| TEXAS INSTRUMENTS INCORPORATED
| Standard Linear and Logic Group
| IBIS Model of SN74LVC14A
| HEX SCHMITT-TRIGGER INVERTERS
| This file contains package information for the following:
|  SOIC 14-pin (D) package as [Component] LVC14A_D
|  SSOP 14-pin (DB) package as [Component] LVC14A_DB
|  TVSOP 14-pin (DGV) package as [Component] LVC14A_DGV
|  SOP 14-pin (NS) package as [Component] LVC14A_NS
|  TSSOP 14-pin (PW) package as [Component] LVC14A_PW
|  QFN 14-pin (RGY) package as [Component] LVC14A_RGY
| This device can be powered at the following Vccs:
|  1.8 volt Vcc
|  2.5 volt Vcc
|  3.3 volt Vcc
|  2.7 volt Vcc
| This file provides unique models under the [Model Selector] for each Vcc.
| For operation at a specific Vcc, select the appropriate model after each
| [Model Selector] keyword.
[IBIS Ver]   3.2
[Comment char]  |_char
[File Name]   sn74lvc14a.ibs
[File Rev]   1.1 | k_die
[Date]   March 31, 2004
[Source]   Data created from TI-SPICE simulations at TI-SLL.
[Notes]   The following is an IBIS list for the LVC14A.
   Please contact sllibis@ti.com with questions and
   comments concerning SLL IBIS models.
   - FILE REV HISTORY
   - 1.1 Release IBIS file on 04/01/04
   - Power clamp data deleted as there is no power-clamp diode.
[Disclaimer] Property of Texas Instruments Incorporated.  Unauthorized
   reproduction and/or distribution is strictly prohibited.
   This product is protected under copyright law.
   Created  2004, (C) Copyright  2004, Texas Instruments
   Incorporated, All Rights Reserved
   UNLESS THERE IS A SIGNED, WRITTEN AGREEMENT TO THE
   CONTRARY, TEXAS INSTRUMENTS (TI) IS PROVIDING THE IBIS
   MODELS  AND WITHOUT ANY WARRANTY, EXPRESSED OR
   IMPLIED.  TI assumes no liability for:
   1) the accuracy of the IBIS models provided to your
   company;
   2) the proper functioning of these IBIS Models in your
   design or for any resulting applications; or
   3) infringement of patents, copyrights or intellectual
   property rights resulting from your use of these IBIS
   models.
   TI provides IBIS Models as a service to our customers.
   You and your company shall not distribute, sell or give
   these models to anyone else without prior written
   permission from TI.
   TI reserves the right to make changes to our products or
   to discontinue any semiconductor product or service
   without notice, and advises our customers to obtain the
   latest version of relevant information to verify, before
   placing orders, that the information being relied on is
   current.
   Please be aware that your receipt and use of the IBIS
   information provided shall serve as acceptance of these
   terms and conditions.  If you do not accept these terms,
   you should return or destroy the IBIS models and any
   other accompanying information immediately.
| Component LVC14A_D 14-pin SOIC
[Component]   LVC14A_D
[Manufacturer]   Texas Instruments, Inc.
[Package]
|   typ   min   max
R_pkg   3.100e-02   2.800e-02   3.400e-02
L_pkg   3.109e-09   2.462e-09   3.889e-09
C_pkg   4.730e-13   3.630e-13   6.280e-13
[Pin]   signal_name   model_name   R_pin   L_pin   C_pin
1   1A   LVC14A_IN   3.300e-02   3.854e-09   6.220e-13
2   1Y   LVC14A_OUT   3.200e-02   3.188e-09   4.730e-13
3   2A   LVC14A_IN   2.800e-02   2.462e-09   3.770e-13
4   2Y   LVC14A_OUT   3.100e-02   2.596e-09   3.630e-13
5   3A   LVC14A_IN   2.800e-02   2.521e-09   3.720e-13
6   3Y   LVC14A_OUT   3.400e-02   3.250e-09   4.760e-13
7   GND   GND   3.400e-02   3.889e-09   6.280e-13
8   4Y   LVC14A_OUT   3.400e-02   3.889e-09   6.280e-13
9   4A   LVC14A_IN   3.400e-02   3.250e-09   4.760e-13
10   5Y   LVC14A_OUT   2.800e-02   2.521e-09   3.720e-13
11   5A   LVC14A_IN   3.100e-02   2.596e-09   3.640e-13
12   6Y   LVC14A_OUT   2.800e-02   2.462e-09   3.770e-13
13   6A   LVC14A_IN   3.200e-02   3.188e-09   4.730e-13
14   VCC   POWER   3.300e-02   3.854e-09   6.220e-13
| Component LVC14A_DB 14-pin SSOP
[Component]   LVC14A_DB
[Manufacturer]   Texas Instruments, Inc.
[Package]
|   typ   min   max
R_pkg   4.400e-02   4.100e-02   4.600e-02
L_pkg   3.551e-09   3.258e-09   3.927e-09
C_pkg   4.020e-13   3.600e-13   4.210e-13
[Pin]   signal_name   model_name   R_pin   L_pin   C_pin
1   1A   LVC14A_IN   4.600e-02   3.927e-09   4.080e-13
2   1Y   LVC14A_OUT   4.400e-02   3.587e-09   4.210e-13
3   2A   LVC14A_IN   4.100e-02   3.289e-09   3.980e-13
4   2Y   LVC14A_OUT   4.200e-02   3.258e-09   3.600e-13
5   3A   LVC14A_IN   4.100e-02   3.286e-09   4.030e-13
6   3Y   LVC14A_OUT   4.400e-02   3.586e-09   4.210e-13
7   GND   GND   4.600e-02   3.927e-09   4.080e-13
8   4Y   LVC14A_OUT   4.600e-02   3.927e-09   4.080e-13
9   4A   LVC14A_IN   4.400e-02   3.586e-09   4.210e-13
10   5Y   LVC14A_OUT   4.100e-02   3.286e-09   4.030e-13
11   5A   LVC14A_IN   4.300e-02   3.258e-09   3.600e-13
12   6Y   LVC14A_OUT   4.100e-02   3.289e-09   3.980e-13
13   6A   LVC14A_IN   4.400e-02   3.587e-09   4.210e-13
14   VCC   POWER   4.600e-02   3.927e-09   4.080e-13
| Component LVC14A_DGV 14-pin TVSOP
[Component]   LVC14A_DGV
[Manufacturer]   Texas Instruments, Inc.
[Package]
|   typ   min   max
R_pkg   3.500e-02   2.000e-02   4.500e-02
L_pkg   2.499e-09   2.077e-09   2.966e-09
C_pkg   3.610e-13   3.050e-13   4.160e-13
[Pin]   signal_name   model_name   R_pin   L_pin   C_pin
1   1A   LVC14A_IN   2.700e-02   2.717e-09   3.730e-13
2   1Y   LVC14A_OUT   3.700e-02   2.434e-09   3.980e-13
3   2A   LVC14A_IN   3.400e-02   2.200e-09   3.160e-13
4   2Y   LVC14A_OUT   2.000e-02   2.077e-09   3.090e-13
5   3A   LVC14A_IN   3.000e-02   2.147e-09   3.050e-13
6   3Y   LVC14A_OUT   4.200e-02   2.580e-09   4.080e-13
7   GND   GND   3.900e-02   2.921e-09   3.850e-13
8   4Y   LVC14A_OUT   3.300e-02   2.841e-09   3.800e-13
9   4A   LVC14A_IN   4.200e-02   2.611e-09   4.100e-13
10   5Y   LVC14A_OUT   3.800e-02   2.331e-09   3.290e-13
11   5A   LVC14A_IN   2.600e-02   2.223e-09   3.190e-13
12   6Y   LVC14A_OUT   3.400e-02   2.259e-09   3.130e-13
13   6A   LVC14A_IN   4.500e-02   2.681e-09   4.160e-13
14   VCC   POWER   4.200e-02   2.966e-09   3.860e-13
| Component LVC14A_NS 14-pin SOP
[Component]   LVC14A_NS
[Manufacturer]   Texas Instruments, Inc.
[Package]
|   typ   min   max
R_pkg   4.500e-02   3.900e-02   5.400e-02
L_pkg   3.796e-09   2.561e-09   4.952e-09
C_pkg   5.280e-13   2.880e-13   7.100e-13
[Pin]   signal_name   model_name   R_pin   L_pin   C_pin
1   1A   LVC14A_IN   4.700e-02   4.867e-09   7.060e-13
2   1Y   LVC14A_OUT   5.100e-02   4.083e-09   5.920e-13
3   2A   LVC14A_IN   4.100e-02   2.915e-09   3.760e-13
4   2Y   LVC14A_OUT   3.900e-02   2.561e-09   2.880e-13
5   3A   LVC14A_IN   4.100e-02   3.101e-09   4.300e-13
6   3Y   LVC14A_OUT   4.700e-02   4.047e-09   5.890e-13
7   GND   GND   5.100e-02   4.909e-09   7.000e-13
8   4Y   LVC14A_OUT   4.500e-02   4.784e-09   6.940e-13
9   4A   LVC14A_IN   5.400e-02   4.176e-09   5.970e-13
10   5Y   LVC14A_OUT   3.900e-02   3.287e-09   4.490e-13
11   5A   LVC14A_IN   3.900e-02   2.586e-09   2.940e-13
12   6Y   LVC14A_OUT   4.000e-02   2.802e-09   3.710e-13
13   6A   LVC14A_IN   4.900e-02   4.080e-09   5.930e-13
14   VCC   POWER   5.200e-02   4.952e-09   7.100e-13
| Component LVC14A_PW 14-pin TSSOP
[Component]   LVC14A_PW
[Manufacturer]  Texas Instruments, Inc.
[Package]
|   typ   min   max
R_pkg   3.200e-02   2.900e-02   3.500e-02
L_pkg   2.378e-09   2.170e-09   2.680e-09
C_pkg   3.140e-13   2.700e-13   3.350e-13
[Pin]   signal_name   model_name   R_pin   L_pin   C_pin
1   1A   LVC14A_IN   3.300e-02   2.618e-09   3.300e-13
2   1Y   LVC14A_OUT   3.100e-02   2.313e-09   3.170e-13
3   2A   LVC14A_IN   3.000e-02   2.310e-09   3.140e-13
4   2Y   LVC14A_OUT   3.100e-02   2.173e-09   2.720e-13
5   3A   LVC14A_IN   3.000e-02   2.204e-09   3.090e-13
6   3Y   LVC14A_OUT   3.200e-02   2.315e-09   3.170e-13
7   GND   GND   3.500e-02   2.680e-09   3.350e-13
8   4Y   LVC14A_OUT   3.300e-02   2.640e-09   3.330e-13
9   4A   LVC14A_IN   3.400e-02   2.347e-09   3.190e-13
10   5Y   LVC14A_OUT   2.900e-02   2.277e-09   3.130e-13
11   5A   LVC14A_IN   3.100e-02   2.170e-09   2.700e-13
12   6Y   LVC14A_OUT   3.100e-02   2.244e-09   3.110e-13
13   6A   LVC14A_IN   3.300e-02   2.343e-09   3.210e-13
14   VCC   POWER   3.500e-02   2.657e-09   3.320e-13
| Component LVC14A_RGY 14-pin QFN
[Component]   LVC14A_RGY
[Manufacturer]   Texas Instruments, Inc.
[Package]
|   typ   min   max
R_pkg   3.200e-02   2.600e-02   4.200e-02
L_pkg   7.210e-10   5.970e-10   9.420e-10
C_pkg   3.110e-13   2.980e-13   3.330e-13
[Pin]   signal_name   model_name   R_pin   L_pin   C_pin
1   1A   LVC14A_IN   3.500e-02   7.880e-10   3.040e-13
2   1Y   LVC14A_OUT   3.700e-02   8.320e-10   3.160e-13
3   2A   LVC14A_IN   4.200e-02   9.420e-10   3.330e-13
4   2Y   LVC14A_OUT   3.100e-02   7.090e-10   3.140e-13
5   3A   LVC14A_IN   3.100e-02   7.080e-10   3.140e-13
6   3Y   LVC14A_OUT   3.200e-02   7.280e-10   3.150e-13
7   GND   GND   3.200e-02   7.200e-10   3.150e-13
8   4Y   LVC14A_OUT   2.600e-02   5.970e-10   2.980e-13
9   4A   LVC14A_IN   3.500e-02   7.920e-10   3.090e-13
10   5Y   LVC14A_OUT   2.800e-02   6.420e-10   3.070e-13
11   5A   LVC14A_IN   2.700e-02   6.130e-10   3.070e-13
12   6Y   LVC14A_OUT   2.800e-02   6.420e-10   3.090e-13
13   6A   LVC14A_IN   3.000e-02   6.760e-10   3.110e-13
14   VCC   POWER   3.100e-02   7.040e-10   3.050e-13
| Model LVC14A_IN
[Model Selector]   LVC14A_IN
LVC14A_IN_18   1.8 volt Vcc
LVC14A_IN_25   2.5 volt Vcc
LVC14A_IN_33   3.3 volt Vcc
LVC14A_IN_27   2.7 volt Vcc
| Model LVC14A_OUT
[Model Selector]   LVC14A_OUT
LVC14A_OUT_18   1.8 volt Vcc
LVC14A_OUT_25   2.5 volt Vcc
LVC14A_OUT_33   3.3 volt Vcc
LVC14A_OUT_27   2.7 volt Vcc
| Models and submodels in the file (8): LVC14A_IN_18 (Input), LVC14A_IN_25 (Input), LVC14A_IN_33 (Input), LVC14A_IN_27 (Input), LVC14A_OUT_18 (Output), LVC14A_OUT_25 (Output), LVC14A_OUT_33 (Output), LVC14A_OUT_27 (Output)
